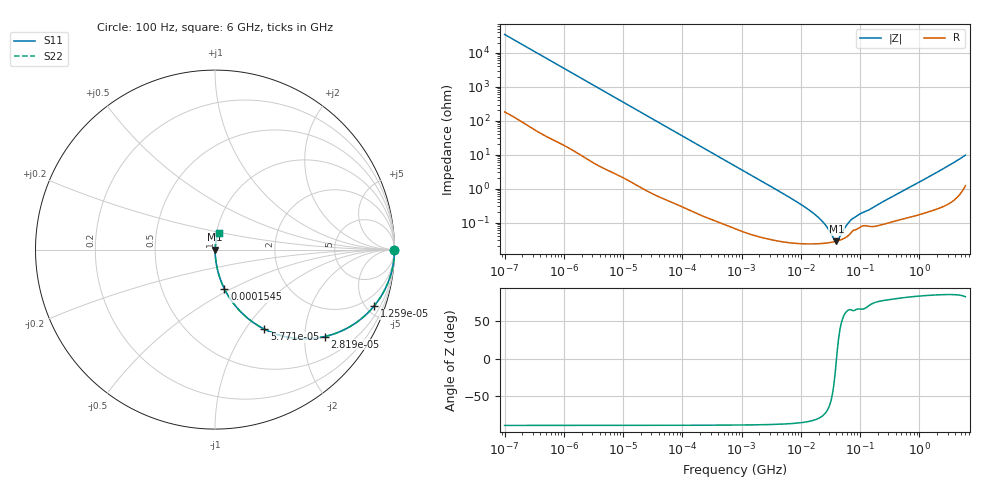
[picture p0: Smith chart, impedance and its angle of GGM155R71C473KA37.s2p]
!Murata Part Number: GGM155R71C473KA37
!These Parameters are Measured in Series Mode Connection
!Data Generated on Jun 19, 2026
!  o--ll--o
!Port1  Port2
!  o------o
!Operation Temp=25[degC], DC Bias Voltage=0[V]
!Freq. Start=100[Hz] Stop=6[GHz] 401[Steps]
# Hz S RI R 50
!Freq.(Hz) S11(Real) S11(Imag) S21(Real) S21(Imag) S12(Real) S12(Imag) S22(Real) S22(Imag)
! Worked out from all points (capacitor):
!   401 points, 100 Hz to 6 GHz, reference 50 ohm
!   read as one part in series: C = 45.8 nF near 109 Hz
!   lowest |Z| = 28.2 mohm at 39.84 MHz (marker M1)
!   series resonance near 40.08 MHz, so ESL is about 340 pH
!   S11 on the Smith chart (normalised r, x): 100 Hz: open; 12.59 kHz: 1.03, -5.60; 28.19 kHz: 1.02, -2.51; 57.71 kHz: 1.01, -1.23; 154.5 kHz: 1.00, -0.46; 6 GHz: 1.02, +0.19
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100  1 -0.00288  2.34e-05 0.00288  2.34e-05 0.00288  1 -0.00288
2008  0.9964 -0.0571  0.00357 0.0571  0.00357 0.0571  0.9964 -0.0571
5378  0.9764 -0.1492  0.0236 0.1492  0.0236 0.1492  0.9764 -0.1492
12592  0.8855 -0.3154  0.1145 0.3154  0.1145 0.3154  0.8855 -0.3154
18841  0.7772 -0.4131  0.2228 0.4131  0.2228 0.4131  0.7772 -0.4131
28191  0.6109 -0.4845  0.3891 0.4845  0.3891 0.4845  0.6109 -0.4845
40335  0.4358 -0.4926  0.5642 0.4926  0.5642 0.4926  0.4358 -0.4926
57709  0.2756 -0.4432  0.7244 0.4432  0.7244 0.4432  0.2756 -0.4432
90302  0.1361 -0.3389  0.8639 0.3389  0.8639 0.3389  0.1361 -0.3389
154540  0.0522 -0.2181  0.9478 0.2181  0.9478 0.2181  0.0522 -0.2181
316350  0.0138 -0.1113  0.9862 0.1113  0.9862 0.1113  0.0138 -0.1113
774597  0.00281 -0.0463  0.9972 0.0463  0.9972 0.0463  0.00281 -0.0463
6353432  0.000286 -0.00559  0.9997 0.00559  0.9997 0.00559  0.000286 -0.00559
1.555665e7  0.000239 -0.00199  0.9998 0.00199  0.9998 0.00199  0.000239 -0.00199
2.434276e7  0.000245 -0.000947  0.9998 0.000947  0.9998 0.000947  0.000245 -0.000947
3.64232e7  0.000271 -0.000175  0.9997 0.000175  0.9997 0.000175  0.000271 -0.000175
3.983537e7  0.000282 -1.09e-05  0.9997 1.09e-05  0.9997 1.09e-05  0.000282 -1.09e-05
4.35672e7  0.000295 0.000153  0.9997 -0.000153  0.9997 -0.000153  0.000295 0.000153
6.233367e7  0.000403 0.000844  0.9996 -0.000844  0.9996 -0.000844  0.000403 0.000844
7.455971e7  0.000564 0.00118  0.9994 -0.00118  0.9994 -0.00118  0.000564 0.00118
3.124326e8  0.00103 0.00511  0.999 -0.00511  0.999 -0.00511  0.00103 0.00511
6e9  0.0208 0.0927  0.9792 -0.0927  0.9792 -0.0927  0.0208 0.0927
